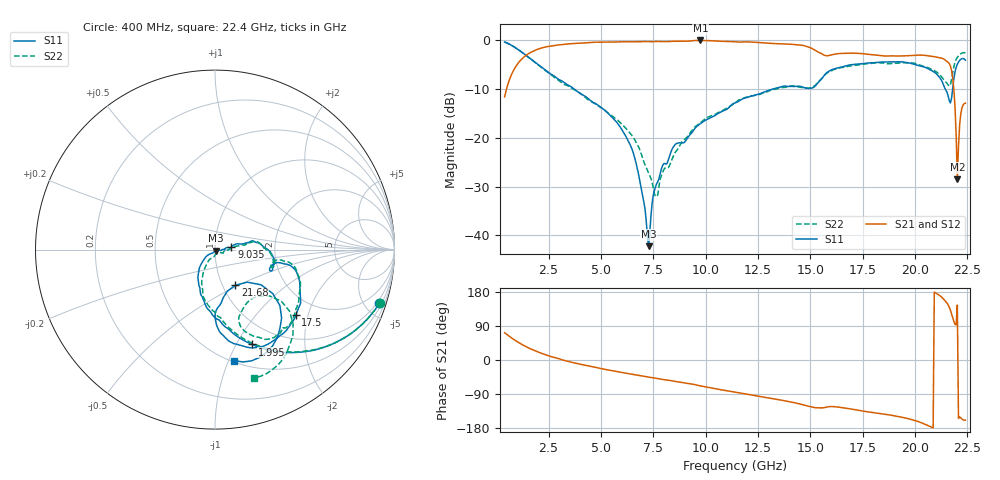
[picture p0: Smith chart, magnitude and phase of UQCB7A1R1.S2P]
!  Part Number  UQCB7A1R1  Mounting Orientation: Vertical
!  Description: RF capacitors
!  Application: Coupling, Bypass, Tuning, DC Block
!  Filters, Matching
# GHZ S DB R 50
! Freq  |S11|  S11 Ph  |S21|  S21 Ph  |S12|  S12 Ph  |S22|  S22 Ph
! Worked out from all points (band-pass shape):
!   401 points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, 400 MHz to 22.4 GHz, reference 50 ohm
!   highest |S21| = 0.00 dB at 9.75 GHz (marker M1); lowest = -28.5 dB at 22.02 GHz (marker M2)
!   |S21| within 3 dB of the highest: 1.439 GHz to 15.65 GHz (14.21 GHz wide, 166 % of centre); 15.96 GHz to 18.15 GHz (2.19 GHz wide, 12.8 % of centre)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
!   lowest |S11| = -42.2 dB at 7.275 GHz (marker M3), VSWR 1.02, Z = 50.4 - j0.656 ohm
!   |S11| at or under -10 dB: 3.729 GHz to 13.18 GHz (9.449 GHz wide, 112 % of centre); 21.45 GHz to 21.79 GHz (344.8 MHz wide, 1.59 % of centre)
!   |S22| runs from -32.0 to -0.3 dB; largest |S21 - S12| = 0.005
!   S11 on the Smith chart (normalised r, x): 400 MHz: 0.76, -6.22; 1.995 GHz: 0.75, -1.16; 9.035 GHz: 1.20, +0.04; 17.5 GHz: 1.53, -1.67; 21.68 GHz: 1.15, -0.48; 22.4 GHz: 0.51, -1.05
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0.4  -0.33 -18.0  -11.59 71.9  -11.61 71.9  -0.32 -17.9
1.115  -2.07 -45.3  -4.30 44.6  -4.31 44.6  -2.08 -45.0
1.995  -4.92 -68.6  -1.78 21.1  -1.79 21.2  -5.00 -68.2
4.085  -11.06 -104.0  -0.53 -12.0  -0.54 -11.9  -11.11 -102.5
6.34  -20.93 -136.7  -0.27 -36.2  -0.26 -36.1  -18.76 -118.8
6.725  -26.06 -141.9  -0.27 -39.9  -0.26 -39.8  -21.22 -120.3
7.275  -42.20 -56.9  -0.24 -45.2  -0.23 -45.0  -27.19 -103.0
7.605  -30.04 -8.3  -0.22 -48.0  -0.21 -47.9  -32.04 -68.3
7.77  -28.35 -1.0  -0.20 -49.7  -0.19 -49.6  -29.98 -30.4
8.485  -21.67 6.8  -0.17 -56.1  -0.16 -55.9  -23.42 -2.6
9.035  -20.63 10.6  -0.17 -60.9  -0.15 -60.8  -20.16 4.7
9.75  -17.04 13.0  0.00 -68.3  -0.01 -68.2  -16.86 9.2
11.4  -12.82 10.4  -0.27 -84.8  -0.26 -84.8  -12.81 11.5
15.085  -9.76 -16.3  -1.67 -124.4  -1.66 -124.5  -9.63 -12.4
15.965  -6.12 -19.1  -2.99 -122.8  -2.99 -123.1  -6.32 -16.8
17.505  -4.75 -38.9  -2.72 -134.8  -2.71 -134.8  -4.89 -38.7
18.77  -4.42 -53.5  -3.18 -144.8  -3.15 -145.1  -4.76 -49.2
20.97  -6.67 -86.3  -3.38 177.5  -3.35 177.2  -6.32 -70.1
21.41  -9.73 -87.7  -3.94 157.5  -3.93 157.3  -8.29 -68.6
21.685  -12.82 -60.4  -5.26 131.6  -5.22 131.3  -9.05 -47.2
22.015  -4.89 -50.5  -28.46 145.1  -28.52 144.8  -3.47 -51.3
22.4  -4.05 -80.2  -12.86 -158.6  -12.83 -158.8  -2.53 -73.3
